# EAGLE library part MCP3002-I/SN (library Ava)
Dual Channel 10-Bit A/D Converter
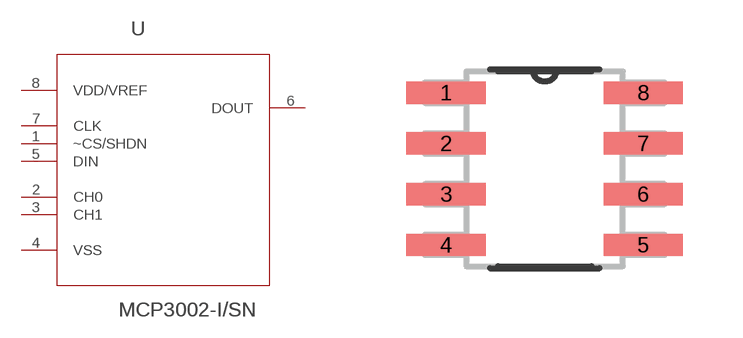
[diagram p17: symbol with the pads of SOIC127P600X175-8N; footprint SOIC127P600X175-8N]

Designator prefix -

## MCP3002-I/SN (DESCRIPTION: Dual Channel 10-Bit A/D Converter; MPN: MCP3002-I/SN; OC_FARNELL: 1834969; OC_NEWARK: 59K0225; PACKAGE: SOIC-8; SUPPLIER: Microchip)  [SOIC127P600X175-8N]
1  ~CS/SHDN  in
2  CH0  in
3  CH1  in
4  VSS  pwr
5  DIN  in
6  DOUT  out
7  CLK  in
8  VDD/VREF  pwr

## Footprint SOIC127P600X175-8N (pad centres in mm)
smd 1.981 x 0.559: 1 -2.464,1.905; 2 -2.464,0.635; 3 -2.464,-0.635; 4 -2.464,-1.905; 5 2.464,-1.905; 6 2.464,-0.635; 7 2.464,0.635; 8 2.464,1.905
